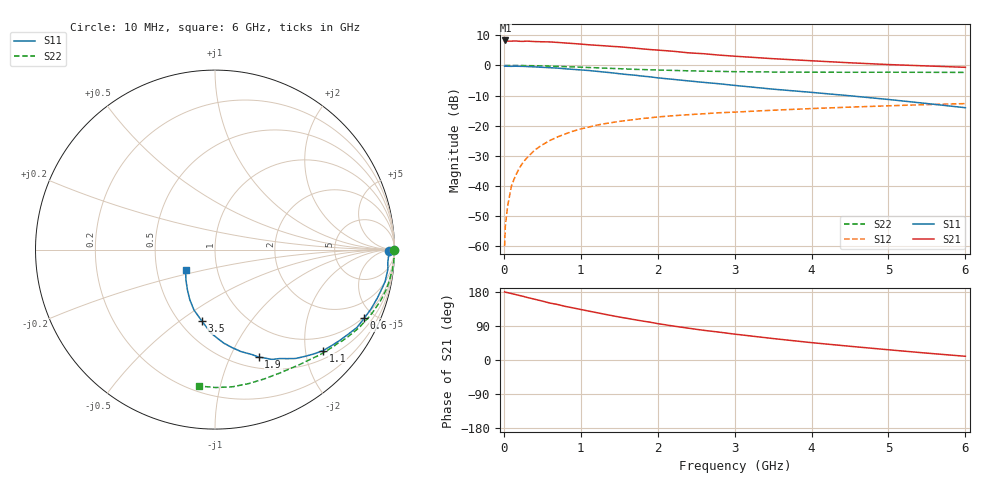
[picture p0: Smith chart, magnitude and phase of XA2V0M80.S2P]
! SIEMENS Discrete & RF Semiconductors
! BFY180
! Si NPN RF Bipolar Junction Transistor in MICRO-X
! VCE = 2 V  IC = 0.8 mA
! Common Emitter S-Parameters:  May  1997
# GHz  S  MA  R  50
!  f  S11  S21  S12  S22
! GHz  MAG  ANG  MAG  ANG  MAG  ANG  MAG  ANG
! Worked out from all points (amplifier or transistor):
!   36 points, 10 MHz to 6 GHz, reference 50 ohm
!   highest |S21| = 8.3 dB at 20 MHz (marker M1)
!   |S21| within 3 dB of that: start of sweep to 1.891 GHz
!   unconditionally stable (mu >= 1): 4.021 GHz to end of sweep
!   at 250 MHz: K = 0.07, MSG = 20.1 dB, |S12| = -32.2 dB
!   at 1.4 GHz: K = 0.48, MSG = 12.7 dB, |S12| = -19.0 dB
!   at 6 GHz: K = 1.06, MAG = 4.5 dB, |S12| = -12.7 dB
!   S11 on the Smith chart (normalised r, x): 10 MHz: 61, -14; 600 MHz: 0.93, -4.38; 1.1 GHz: 0.68, -2.37; 1.9 GHz: 0.62, -1.29; 3.5 GHz: 0.64, -0.60; 6 GHz: 0.70, -0.17
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0.01  0.9693 -0.4  2.516 179.7  0.001 85.5  0.9985 -0.1
0.02  0.9723 -0.7  2.595 178.9  0.0022 91.2  0.9984 -0.5
0.05  0.9674 -2.3  2.532 177.7  0.0047 87.1  0.9979 -1.2
0.1  0.9656 -4.2  2.527 175.3  0.0101 89.8  0.9983 -2.6
0.15  0.9696 -6.6  2.548 172.9  0.0146 86.0  0.9979 -3.9
0.2  0.9665 -8.4  2.515 170.4  0.0196 84.8  0.9953 -5.1
0.3  0.9579 -12.4  2.532 165.2  0.0293 81.2  0.9909 -7.7
0.4  0.9444 -16.5  2.487 160.4  0.0392 78.7  0.987 -10.2
0.6  0.9155 -24.7  2.454 150.2  0.0569 72.6  0.9728 -15.0
0.8  0.8782 -32.6  2.356 141.4  0.073 66.6  0.9536 -19.7
1.1  0.8239 -43.1  2.202 129.2  0.0945 59.1  0.923 -26.1
1.3  0.7764 -50.1  2.118 121.2  0.1073 54.5  0.9022 -30.2
1.5  0.7285 -56.5  2.037 113.4  0.1177 50.4  0.8821 -34.0
1.9  0.6467 -67.9  1.833 99.8  0.1349 43.6  0.846 -40.6
2.2  0.587 -75.6  1.718 89.7  0.1461 39.2  0.8261 -45.4
2.6  0.5229 -84.7  1.563 78.3  0.1577 34.5  0.8028 -51.0
3  0.4659 -92.7  1.422 68.3  0.1678 30.3  0.7874 -56.4
3.5  0.4035 -100.6  1.293 56.6  0.1805 26.0  0.7761 -62.7
4  0.357 -109.1  1.194 45.8  0.1922 21.7  0.7709 -69.2
4.5  0.3131 -116.6  1.105 36.2  0.2032 17.5  0.7698 -75.8
5.5  0.233 -134.1  0.98 18.1  0.2237 9.5  0.7686 -89.7
6  0.1986 -145.2  0.93 9.8  0.2324 5.1  0.7654 -96.7
